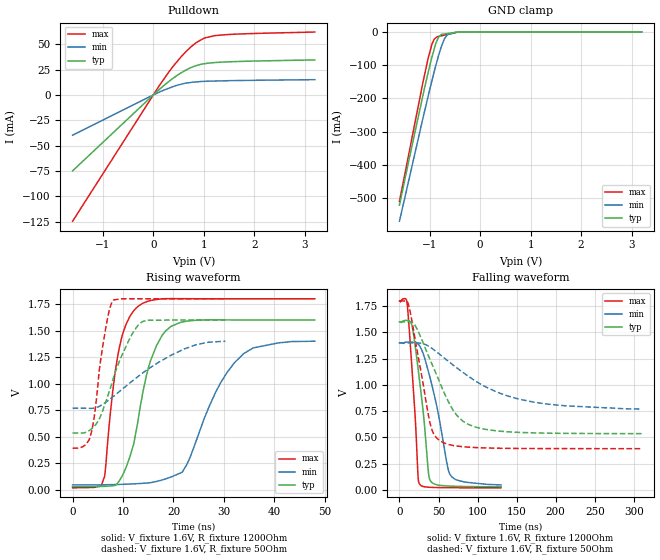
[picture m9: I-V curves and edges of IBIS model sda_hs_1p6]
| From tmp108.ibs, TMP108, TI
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|   sda_hs_1p6 Model
[Model]   sda_hs_1p6
Model_type   I/O_open_drain
Polarity   Non-Inverting
Vinl = 0.5
Vinh = 1.4
Vmeas = 0.8
Vref = 1.6
Cref = 2pF
Rref = 1200
|   typ   min   max
C_comp   9.450e-13   9.305e-13   9.710e-13
| Where nom  PVT is Nominal Process, 1.6V, 27C
|   Fast PVT is Strong Process,  1.8V, -40C
|   Slow PVT is Weak Process,   1.4V, 125C
[Voltage Range]   1.6   1.4   1.8
|Ambient Temperature   25   125   -40
|Junction Temperature
[Temperature Range]   27   125   -40
[Pullup Reference]   1.6   1.4   1.8
[Pulldown Reference]   0   0   0
[Power Clamp Reference]   1.6   1.4   1.8
[GND Clamp Reference]   0   0   0
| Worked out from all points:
|   slope of the pulldown table from 0 to 0.24 V, typ, clamps not added: 22.7 ohm
|   GND clamp passes 1 mA (typ) near -0.49 V on its own axis
|   falling waveform, V_fixture 1.6V, R_fixture 1200Ohm: 20-80 % time 13.4ns typ, 22.2ns min, 8.91ns max; typ from 1.6 V to 0.028 V
|   rising waveform, V_fixture 1.6V, R_fixture 1200Ohm: 20-80 % time 4.48ns typ, 7.61ns min, 2.96ns max; typ from 0.028 V to 1.6 V
|   falling waveform, V_fixture 1.6V, R_fixture 50Ohm: 20-80 % time 38.7ns typ, 83.7ns min, 19.9ns max; typ from 1.6 V to 0.535 V
|   rising waveform, V_fixture 1.6V, R_fixture 50Ohm: 20-80 % time 4.94ns typ, 11.3ns min, 2.31ns max; typ from 0.535 V to 1.6 V
[Pulldown]
|   Voltage   I(typ)   I(min)   I(max)
-1.6V     -74.82mA   -39.68mA   -124.5mA
126mV     5.698mA    2.974mA    9.698mA
394.2mV   16.52mA    8.24mA     28.27mA
612mV     23.57mA    11.31mA    40.9mA
777.6mV   27.6mA     12.64mA    48.7mA
862.2mV   29.08mA    12.86mA    51.96mA
1.008V    30.76mA    13.41mA    55.97mA
1.238V    31.97mA    13.74mA    58.55mA
1.699V    32.99mA    14.22mA    60.05mA
3.2V      34.52mA    15.06mA    61.98mA
[GND Clamp]
|   Voltage   I(typ)   I(min)   I(max)
-1.6V     -521mA     -569.6mA   -510mA
-1.132V   -189.1mA   -258mA     -150mA
-1.028V   -120.1mA   -191.1mA   -77.06mA
-955.8mV  -75.43mA   -146.4mA   -36.66mA
-909mV    -50.02mA   -118.5mA   -21.14mA
-880mV    -34.58mA   -101.3mA   -17.55mA
-828.8mV  -16.42mA   -72.81mA   -13.38mA
-771.2mV  -7.324mA   -44.62mA   -11.36mA
-711.2mV  -5.968mA   -21.37mA   -9.266mA
-651mV    -4.608mA   -7.937mA   -7.161mA
-428.4mV  -33.37uA   -90.99uA   -36.31uA
3.2V      0A         0A         0A
[POWER Clamp]
|   Voltage   I(typ)   I(min)   I(max)
-1.6V     0A         0A         0A
-1.598V   0A         0A         0A
3.2V      0A         0A         0A
[Ramp]
R_load = 1200
|   typ   min   max
dV/dt_r   0.943088/4.41571e-09   0.812079/7.58273e-09   1.0687/2.95572e-09
dV/dt_f   0.943088/1.3391e-08   0.812073/2.22165e-08   1.0687/8.9099e-09
[Falling Waveform]
V_fixture = 1.6V
V_fixture_min = 1.4V
V_fixture_max = 1.8V
R_fixture = 1200Ohm
|   Time   V(typ)   V(min)   V(max)
0s        1.6V       1.4V       1.8V
9.98ns    1.613V     1.408V     1.767V
16.49ns   1.55V      1.406V     1.104V
20.37ns   1.361V     1.401V     668mV
23.98ns   1.148V     1.388V     109mV
25.27ns   1.069V     1.378V     58.88mV
37.52ns   139.3mV    1.115V     24.51mV
39.65ns   85.2mV     1.053V     23.63mV
64.35ns   35.2mV     150.9mV    20.14mV
130ns     28.19mV    46.54mV    18.83mV
[Rising Waveform]
V_fixture = 1.6V
V_fixture_min = 1.4V
V_fixture_max = 1.8V
R_fixture = 1200Ohm
|   Time   V(typ)   V(min)   V(max)
0s        28.19mV    46.53mV    18.83mV
6.26ns    32.7mV     47.51mV    114.1mV
9.15ns    77.16mV    50.87mV    1.311V
12.93ns   640.2mV    58.44mV    1.726V
15.46ns   1.217V     67.84mV    1.784V
19.52ns   1.54V      120.9mV    1.802V
22.64ns   1.59V      237.6mV    1.801V
28.38ns   1.602V     922.2mV    1.8V
33.91ns   1.6V       1.283V     1.8V
48ns      1.6V       1.4V       1.8V
[Falling Waveform]
V_fixture = 1.6V
V_fixture_min = 1.4V
V_fixture_max = 1.8V
R_fixture = 50Ohm
|   Time   V(typ)   V(min)   V(max)
0s        1.6V       1.4V       1.8V
12.22ns   1.6V       1.4V       1.747V
22.39ns   1.535V     1.4V       1.337V
39.09ns   1.241V     1.36V      638.2mV
44.07ns   1.156V     1.334V     529.9mV
52.07ns   1.014V     1.287V     466mV
73.64ns   708mV      1.161V     416.7mV
101.8ns   588.9mV    1.016V     401.1mV
172.1ns   542.2mV    835.2mV    393.2mV
310ns     535.2mV    769.4mV    392.3mV
[Rising Waveform]
V_fixture = 1.6V
V_fixture_min = 1.4V
V_fixture_max = 1.8V
R_fixture = 50Ohm
|   Time   V(typ)   V(min)   V(max)
0s        535.1mV    769.1mV    392.3mV
3.47ns    563.9mV    767.6mV    496.2mV
4.35ns    601mV      770.8mV    706.6mV
5.26ns    664.5mV    786.1mV    1.113V
6.38ns    802.1mV    818.3mV    1.47V
8.02ns    1.04V      877.4mV    1.785V
11.05ns   1.398V     995.2mV    1.8V
13.89ns   1.585V     1.1V       1.8V
22.13ns   1.6V       1.327V     1.8V
30.3ns    1.6V       1.4V       1.8V
